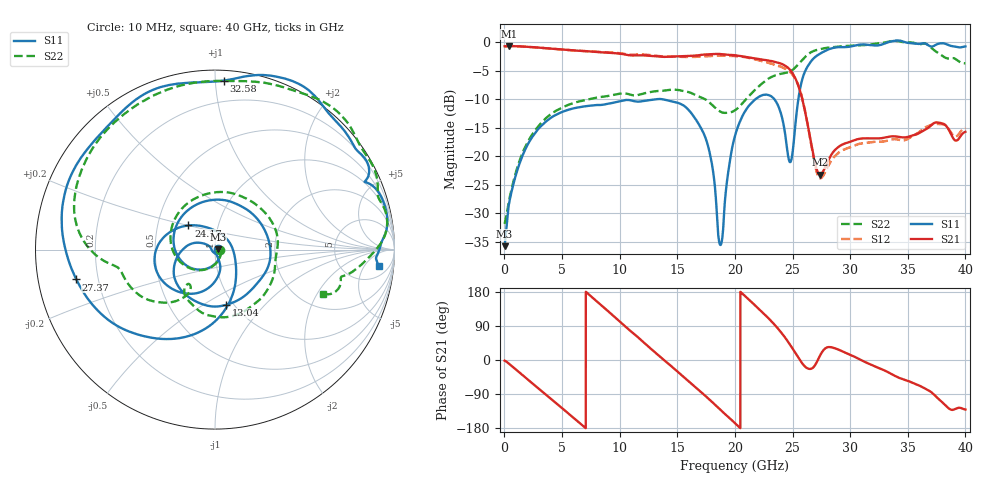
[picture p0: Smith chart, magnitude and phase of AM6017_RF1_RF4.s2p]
!Agilent Technologies,E8364B,MY43040894,A.07.50.67
!Agilent E8364B: A.07.50.67
!Date: Wednesday, July 17, 2019 10:34:54
!Correction: S11(Full 2 Port(1,2))
!S21(Full 2 Port(1,2))
!S12(Full 2 Port(1,2))
!S22(Full 2 Port(1,2))
!S2P File: Measurements: S11, S21, S12, S22:
# Hz S  dB  R 50
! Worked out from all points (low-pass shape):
!   6401 points, 10 MHz to 40 GHz, reference 50 ohm
!   highest |S21| = -0.68 dB at 403.7 MHz (marker M1); lowest = -23.2 dB at 27.38 GHz (marker M2)
!   |S21| within 3 dB of the highest: start of sweep to 23.89 GHz
!   lowest |S11| = -35.8 dB at 10 MHz (marker M3), VSWR 1.03, Z = 51.6 + j0.255 ohm
!   |S11| at or under -10 dB: start of sweep to 13.24 GHz; 13.65 GHz to 21.79 GHz (8.135 GHz wide, 45.9 % of centre); 23.42 GHz to 25.5 GHz (2.086 GHz wide, 8.53 % of centre)
!   |S22| runs from -31.9 to 0.2 dB; largest |S21 - S12| = 0.042
!   S11 on the Smith chart (normalised r, x): 10 MHz: 1.03, +0.01; 13.04 GHz: 0.92, -0.63; 24.17 GHz: 0.72, +0.20; 27.37 GHz: 0.12, -0.10; 32.58 GHz: 0.06, +1.05; 40 GHz: 10, -11
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1e7  -35.78 8.7  -0.72 -1.7  -0.75 -2.1  -31.88 -8.7
4.036516e8  -28.20 -38.0  -0.68 -10.2  -0.67 -10.2  -27.68 -39.2
3.452889e9  -14.17 -159.8  -1.04 -88.0  -1.04 -87.9  -13.60 -162.5
6.677083e9  -11.35 113.4  -1.54 -170.1  -1.54 -170.0  -10.30 111.7
9.963761e9  -10.38 11.2  -2.01 102.3  -1.93 102.3  -9.05 25.6
1.303799e10  -10.05 -79.0  -2.47 20.7  -2.34 19.3  -8.62 -41.7
1.334417e10  -9.98 -86.9  -2.52 12.6  -2.42 11.1  -8.55 -48.1
1.729318e10  -16.02 172.6  -2.18 -90.7  -2.48 -92.1  -9.89 -117.8
1.873032e10  -35.57 -140.6  -2.08 -131.1  -2.35 -131.3  -12.18 -128.5
2.0005e10  -16.42 -83.8  -2.30 -166.8  -2.43 -166.9  -11.94 -122.3
2.231692e10  -9.34 -149.6  -3.04 128.0  -3.30 126.1  -7.32 -137.2
2.417271e10  -13.97 137.8  -3.92 66.5  -4.47 67.0  -5.48 -164.6
2.484754e10  -20.91 26.2  -5.02 37.4  -5.36 39.2  -5.07 -170.2
2.587228e10  -6.30 -103.6  -10.25 -10.3  -10.09 -11.1  -3.05 179.2
2.667208e10  -3.19 -142.4  -18.37 -22.4  -18.57 -26.3  -1.70 162.7
2.736566e10  -2.04 -167.9  -23.21 10.5  -23.86 7.0  -1.23 148.0
2.73844e10  -2.02 -168.5  -23.22 11.6  -23.88 8.2  -1.22 147.7
3.027743e10  -0.66 124.2  -17.25 10.0  -18.22 13.5  -0.58 100.2
3.25831e10  -0.51 87.1  -16.87 -22.5  -17.46 -17.6  -0.18 68.0
3.333917e10  0.02 76.1  -16.58 -32.9  -17.20 -26.8  0.10 57.1
3.650088e10  -0.23 28.6  -15.37 -75.4  -14.96 -68.6  -0.25 9.3
4e10  -0.75 -5.9  -15.71 -130.8  -15.04 -124.9  -3.71 -22.5
